| IBIS file stm32wba52_a54_ufqfpn32.ibs
[IBIS ver] 4.2
[File name] stm32wba52_a54_ufqfpn32.ibs
[File Rev] 1.2
[Date] 22-05-2024
[Source] Data Created at STMicroelectronics
[Notes]  File originated from ELDO simulations.
[Disclaimer]  This information is for modeling purpose only and is
   not guaranteed. The information is subject to change without
   notice.
[Copyright] Copyright 2024 STMicroelectronics Inc.
|   Component stm32wba52_a54_ufqfpn32
[Component] stm32wba52_a54_ufqfpn32
[Manufacturer] STMicroelectronics
[Package]
| variable   typ   min   max
R_pkg  0  NA  NA
L_pkg  0  NA  NA
C_pkg  0  NA  NA
[Pin]   signal_name   model_name
0  VSS  gnd
1  PB12  io8_ft_100m_v33
2  PA8  io8_ft_100m_v33
3  PA7  io8_ft_100m_i2c_v33
4  PA6  io8_ft_100m_i2c_v33
5  VDDA  nc
6  PA5  io8_ft_100m_v33
7  PA2  io8_ft_100m_v33
8  PA1  io8_ft_100m_v33
9  PA0  io8_ft_100m_v33
10  PB9  io8_ft_100m_v33
11  PB8  io8_ft_100m_v33
12  PC15-OSC32_OUT  io8_ft_100m_tamp
13  PC14-OSC32_IN  io8_ft_100m_tamp
14  VDD  power
15  PB4  io8_ft_100m_v33
16  PB3  io8_ft_100m_i2c_v33
17  PA15  io8_ft_100m_i2c_v33
18  PA14  io8_ft_100m_v33
19  PA13  io8_ft_100m_v33
20  PA12  io8_ft_100m_v33
21  PB15  io8_ft_100m_v33
22  PH3-BOOT0  io8_ft_100m_v33
23  VDD  power
24  NRST  ioreset_v33
25  RF  nc
26  VDDHPA  nc
27  VDDRF  nc
28  OSC_OUT  nc
29  OSC_IN  nc
30  VDDRFPA  nc
31  VDD  power
32  VCAP  nc
[Package Model]   492-ufqfpn-5x5-32l-230116
[Pin Mapping]   pulldown_ref   pullup_ref   | Comment
0  gndio  nc
1  gndio  vddiom
2  gndio  vddiom
3  gndio  vddiom
4  gndio  vddiom
5  nc  nc
6  gndio  vddiom
7  gndio  vddiom
8  gndio  vddiom
9  gndio  vddiom
10  gndio  vddiom
11  gndio  vddiom
12  gndio  vddiom
13  gndio  vddiom
14  nc  vddiom
15  gndio  vddiom
16  gndio  vddiom
17  gndio  vddiom
18  gndio  vddiom
19  gndio  vddiom
20  gndio  vddiom
21  gndio  vddiom
22  gndio  vddiom
23  nc  vddiom
24  gndio  vddiom
25  nc  nc
26  nc  nc
27  nc  nc
28  nc  nc
29  nc  nc
30  nc  nc
31  nc  vddiom
32  nc  nc
[Model Selector] io8_ft_100m_i2c_v33
io8_ft_100m_v33_ls_1v2  "GPIO_V33 100MHz - 5V tolerant - low speed - 1.2V range"
io8_ft_100m_v33_ls_1v8  "GPIO_V33 100MHz - 5V tolerant - low speed - 1.8V range"
io8_ft_100m_v33_ls_3v3  "GPIO_V33 100MHz - 5V tolerant - low speed - 3.3V range"
io8_ft_100m_v33_ms_1v2  "GPIO_V33 100MHz - 5V tolerant - med speed - 1.2V range"
io8_ft_100m_v33_ms_1v8  "GPIO_V33 100MHz - 5V tolerant - med speed - 1.8V range"
io8_ft_100m_v33_ms_3v3  "GPIO_V33 100MHz - 5V tolerant - med speed - 3.3V range"
io8_ft_100m_v33_fs_1v2  "GPIO_V33 100MHz - 5V tolerant - fast speed - 1.2V range"
io8_ft_100m_v33_fs_1v8  "GPIO_V33 100MHz - 5V tolerant - fast speed - 1.8V range"
io8_ft_100m_v33_fs_3v3  "GPIO_V33 100MHz - 5V tolerant - fast speed - 3.3V range"
io8_ft_100m_v33_hs_1v2  "GPIO_V33 100MHz - 5V tolerant - high speed - 1.2V range"
io8_ft_100m_v33_hs_1v8  "GPIO_V33 100MHz - 5V tolerant - high speed - 1.8V range"
io8_ft_100m_v33_hs_3v3  "GPIO_V33 100MHz - 5V tolerant - high speed - 3.3V range"
io8_ft_100m_i2c_v33_ls_1v2  "GPIO_V33 100MHz with I2C open-drain - 5V tolerant - low speed - 1.2V range"
io8_ft_100m_i2c_v33_ls_1v8  "GPIO_V33 100MHz with I2C open-drain - 5V tolerant - low speed - 1.8V range"
io8_ft_100m_i2c_v33_ls_3v3  "GPIO_V33 100MHz with I2C open-drain - 5V tolerant - low speed - 3.3V range"
io8_ft_100m_i2c_v33_ms_1v2  "GPIO_V33 100MHz with I2C open-drain - 5V tolerant - med speed - 1.2V range"
io8_ft_100m_i2c_v33_ms_1v8  "GPIO_V33 100MHz with I2C open-drain - 5V tolerant - med speed - 1.8V range"
io8_ft_100m_i2c_v33_ms_3v3  "GPIO_V33 100MHz with I2C open-drain - 5V tolerant - med speed - 3.3V range"
io8_ft_100m_i2c_v33_fs_1v2  "GPIO_V33 100MHz with I2C open-drain - 5V tolerant - fast speed - 1.2V range"
io8_ft_100m_i2c_v33_fs_1v8  "GPIO_V33 100MHz with I2C open-drain - 5V tolerant - fast speed - 1.8V range"
io8_ft_100m_i2c_v33_fs_3v3  "GPIO_V33 100MHz with I2C open-drain - 5V tolerant - fast speed - 3.3V range"
io8_ft_100m_i2c_v33_hs_1v2  "GPIO_V33 100MHz with I2C open-drain - 5V tolerant - high speed - 1.2V range"
io8_ft_100m_i2c_v33_hs_1v8  "GPIO_V33 100MHz with I2C open-drain - 5V tolerant - high speed - 1.8V range"
io8_ft_100m_i2c_v33_hs_3v3  "GPIO_V33 100MHz with I2C open-drain - 5V tolerant - high speed - 3.3V range"
io8_ft_100m_i2c_fmp_v33_3v3  "GPIO_V33 100MHz with I2C fm+ open-drain - 5V tolerant - low speed - 3.3V range"
[Model Selector] io8_ft_100m_tamp
io8_ft_100m_ls_1v2 "GPIO SPI - 5V tolerant - low speed - 1.2V range"
io8_ft_100m_ls_1v8 "GPIO SPI - 5V tolerant - low speed - 1.8V range"
io8_ft_100m_ls_3v3 "GPIO SPI - 5V tolerant - low speed - 3.3V range"
io8_ft_100m_ms_1v2 "GPIO SPI - 5V tolerant - med speed - 1.2V range"
io8_ft_100m_ms_1v8 "GPIO SPI - 5V tolerant - med speed - 1.8V range"
io8_ft_100m_ms_3v3 "GPIO SPI - 5V tolerant - med speed - 3.3V range"
io8_ft_100m_fs_1v2 "GPIO SPI - 5V tolerant - fast speed - 1.2V range"
io8_ft_100m_fs_1v8 "GPIO SPI - 5V tolerant - fast speed - 1.8V range"
io8_ft_100m_fs_3v3 "GPIO SPI - 5V tolerant - fast speed - 3.3V range"
io8_ft_100m_hs_1v2 "GPIO SPI - 5V tolerant - high speed - 1.2V range"
io8_ft_100m_hs_1v8 "GPIO SPI - 5V tolerant - high speed - 1.8V range"
io8_ft_100m_hs_3v3 "GPIO SPI - 5V tolerant - high speed - 3.3V range"
io8_ft_tamp_ls_1v2 "IO TAMPER_3V - 5V tolerant - low speed - 1.2V range"
io8_ft_tamp_ls_1v8 "IO TAMPER_3V - 5V tolerant - low speed - 1.8V range"
io8_ft_tamp_ls_3v3 "IO TAMPER_3V-  5V tolerant - low speed - 3.3V range"
io8_ft_tamp_ms_1v2 "IO TAMPER_3V - 5V tolerant - med speed - 1.2V range"
io8_ft_tamp_ms_1v8 "IO TAMPER_3V - 5V tolerant - med speed - 1.8V range"
io8_ft_tamp_ms_3v3 "IO TAMPER_3V - 5V tolerant - med speed - 3.3V range"
io8_ft_tamp_fs_1v2 "IO TAMPER_3V - 5V tolerant - fast speed - 1.2V range"
io8_ft_tamp_fs_1v8 "IO TAMPER_3V - 5V tolerant - fast speed - 1.8V range"
io8_ft_tamp_fs_3v3 "IO TAMPER_3V - 5V tolerant - fast speed - 3.3V range"
io8_ft_tamp_hs_1v2 "IO TAMPER_3V - 5V tolerant - high speed - 1.2V range"
io8_ft_tamp_hs_1v8 "IO TAMPER_3V - 5V tolerant - high speed - 1.8V range"
io8_ft_tamp_hs_3v3 "IO TAMPER_3V - 5V tolerant - high speed - 3.3V range"
[Model Selector] io8_ft_100m_v33
io8_ft_100m_v33_ls_1v2  "GPIO_V33 100MHz - 5V tolerant - low speed - 1.2V range"
io8_ft_100m_v33_ls_1v8  "GPIO_V33 100MHz - 5V tolerant - low speed - 1.8V range"
io8_ft_100m_v33_ls_3v3  "GPIO_V33 100MHz - 5V tolerant - low speed - 3.3V range"
io8_ft_100m_v33_ms_1v2  "GPIO_V33 100MHz - 5V tolerant - med speed - 1.2V range"
io8_ft_100m_v33_ms_1v8  "GPIO_V33 100MHz - 5V tolerant - med speed - 1.8V range"
io8_ft_100m_v33_ms_3v3  "GPIO_V33 100MHz - 5V tolerant - med speed - 3.3V range"
io8_ft_100m_v33_fs_1v2  "GPIO_V33 100MHz - 5V tolerant - fast speed - 1.2V range"
io8_ft_100m_v33_fs_1v8  "GPIO_V33 100MHz - 5V tolerant - fast speed - 1.8V range"
io8_ft_100m_v33_fs_3v3  "GPIO_V33 100MHz - 5V tolerant - fast speed - 3.3V range"
io8_ft_100m_v33_hs_1v2  "GPIO_V33 100MHz - 5V tolerant - high speed - 1.2V range"
io8_ft_100m_v33_hs_1v8  "GPIO_V33 100MHz - 5V tolerant - high speed - 1.8V range"
io8_ft_100m_v33_hs_3v3  "GPIO_V33 100MHz - 5V tolerant - high speed - 3.3V range"
[Model Selector] ioreset_v33
ioreset_v33_1v2 "Reset PAD. 5V tolerant. 1.2V range"
ioreset_v33_1v8 "Reset PAD. 5V tolerant. 1.8V range"
ioreset_v33_3v3 "Reset PAD. 5V tolerant. 3.3V range"
[Define Package Model]  492-ufqfpn-5x5-32l-230116
[Manufacturer]  Unknown
[OEM]  Unknown
[Description]  None
[Number Of Pins]  33
[Pin Numbers]
| Pin Num   Terminal Name
25 | RF
24 | NRST
9 | PA0
20 | PA12
19 | PA13
18 | PA14
17 | PA15
8 | PA1
7 | PA2
6 | PA5
4 | PA6
3 | PA7
2 | PA8
1 | PB12
21 | PB15
16 | PB3
15 | PB4
11 | PB8
10 | PB9
13 | PC14-OSC32_IN
12 | PC15-OSC32_OUT
22 | PH3-BOOT0
32 | VCAP
31 | VDD
23 | VDD
14 | VDD
5 | VDDA
26 | VDDHPA
27 | VDDRF
30 | VDDRFPA
0 | VSS
29 | OSC_IN
28 | OSC_OUT
[Model Data]
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[End Model Data]
[End Package Model]
|End [Component]
| Models and submodels in the file (52): io8_ft_100m_fs_1v2 (I/O), io8_ft_100m_fs_1v8 (I/O), io8_ft_100m_fs_3v3 (I/O), io8_ft_100m_hs_1v2 (I/O), io8_ft_100m_hs_1v8 (I/O), io8_ft_100m_hs_3v3 (I/O), io8_ft_100m_i2c_fmp_v33_3v3 (I/O_open_drain), io8_ft_100m_i2c_v33_fs_1v2 (I/O_open_drain), io8_ft_100m_i2c_v33_fs_1v8 (I/O_open_drain), io8_ft_100m_i2c_v33_fs_3v3 (I/O_open_drain), io8_ft_100m_i2c_v33_hs_1v2 (I/O_open_drain), io8_ft_100m_i2c_v33_hs_1v8 (I/O_open_drain), io8_ft_100m_i2c_v33_hs_3v3 (I/O_open_drain), io8_ft_100m_i2c_v33_ls_1v2 (I/O_open_drain), io8_ft_100m_i2c_v33_ls_1v8 (I/O_open_drain), io8_ft_100m_i2c_v33_ls_3v3 (I/O_open_drain), io8_ft_100m_i2c_v33_ms_1v2 (I/O_open_drain), io8_ft_100m_i2c_v33_ms_1v8 (I/O_open_drain), io8_ft_100m_i2c_v33_ms_3v3 (I/O_open_drain), io8_ft_100m_ls_1v2 (I/O), io8_ft_100m_ls_1v8 (I/O), io8_ft_100m_ls_3v3 (I/O), io8_ft_100m_ms_1v2 (I/O), io8_ft_100m_ms_1v8 (I/O), io8_ft_100m_ms_3v3 (I/O), io8_ft_100m_v33_fs_1v2 (I/O), io8_ft_100m_v33_fs_1v8 (I/O), io8_ft_100m_v33_fs_3v3 (I/O), io8_ft_100m_v33_hs_1v2 (I/O), io8_ft_100m_v33_hs_1v8 (I/O), io8_ft_100m_v33_hs_3v3 (I/O), io8_ft_100m_v33_ls_1v2 (I/O), io8_ft_100m_v33_ls_1v8 (I/O), io8_ft_100m_v33_ls_3v3 (I/O), io8_ft_100m_v33_ms_1v2 (I/O), io8_ft_100m_v33_ms_1v8 (I/O), io8_ft_100m_v33_ms_3v3 (I/O), io8_ft_tamp_fs_1v2 (I/O), io8_ft_tamp_fs_1v8 (I/O), io8_ft_tamp_fs_3v3 (I/O), io8_ft_tamp_hs_1v2 (I/O), io8_ft_tamp_hs_1v8 (I/O), io8_ft_tamp_hs_3v3 (I/O), io8_ft_tamp_ls_1v2 (I/O), io8_ft_tamp_ls_1v8 (I/O), io8_ft_tamp_ls_3v3 (I/O), io8_ft_tamp_ms_1v2 (I/O), io8_ft_tamp_ms_1v8 (I/O), io8_ft_tamp_ms_3v3 (I/O), ioreset_v33_1v2 (I/O_open_drain), ioreset_v33_1v8 (I/O_open_drain), ioreset_v33_3v3 (I/O_open_drain)
